(* Logix 5000 AddOnInstructionDefinition export AMCI_3601_AOP_Immediate_Stop; software revision 20.03 *)

ADD_ON_INSTRUCTION AMCI_3601_AOP_Immediate_Stop   (* revision 0.0, vendor AMCI, ExecuteEnableInFalse *)
// Revision note:
// 3/2020: Version 0 is the initial release
VAR_INPUT
   Axis_Status_Bits : INT; {required}
END_VAR
VAR_OUTPUT
   EN : BOOL; {access Read Only, visible}
   ER : BOOL; {access Read Only, visible}
END_VAR
VAR_IN_OUT
   AMCI_3601_output_data : AM:1769_3601:O:0; {required}
END_VAR
VAR
   Upper_Result_X_1000 : DINT;
   command_data_block : INT[10];
        [0]   // Command Bits MSW
        [1]   // Command Bits LSW
        [2]   // Upper Target Position
        [3]   // Lower Target Position
        [4]   // Upper Programmed Speed
        [5]   // Lower Programmed Speed
END_VAR

ROUTINE EnableInFalse   (* ladder *)
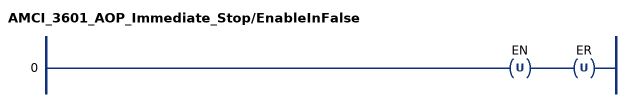
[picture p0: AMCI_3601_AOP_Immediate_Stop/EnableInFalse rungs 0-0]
   0: OTU(EN)OTU(ER);
END_ROUTINE

ROUTINE Logic   (* ladder *)
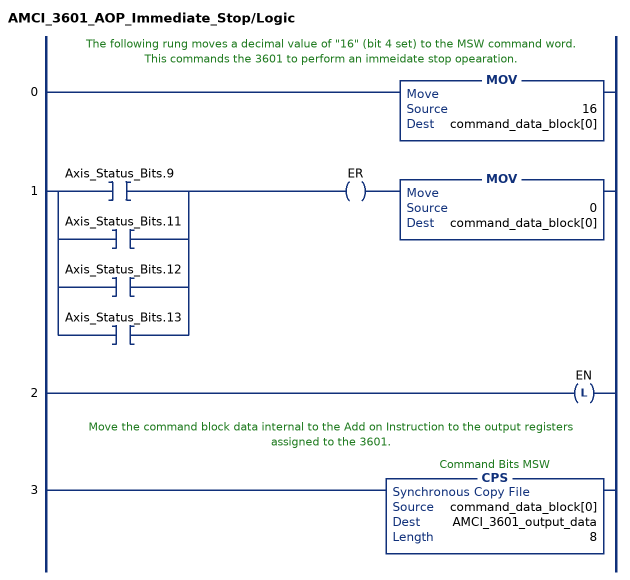
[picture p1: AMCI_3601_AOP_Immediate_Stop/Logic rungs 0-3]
   // The following rung moves a decimal value of "16" (bit 4 set) to the MSW command word.  This commands the 3601 to perform an immeidate stop opearation.
   0: MOV(16,command_data_block[0]);
   1: [XIC(Axis_Status_Bits.9) ,XIC(Axis_Status_Bits.11) ,XIC(Axis_Status_Bits.12) ,XIC(Axis_Status_Bits.13) ]OTE(ER)MOV(0,command_data_block[0]);
   2: OTL(EN);
   // Move the command block data internal to the Add on Instruction to the output registers assigned to the 3601.
   3: CPS(command_data_block[0],AMCI_3601_output_data,8);
END_ROUTINE
END_ADD_ON_INSTRUCTION
